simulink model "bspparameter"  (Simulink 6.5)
settings: Solver=ode45  SolverMode=SingleTasking  StartTime=0.0  StopTime=500.0  FixedStep=0.01  RelTol=1e-3
PostLoadFcn:
  | bspparameter_ini
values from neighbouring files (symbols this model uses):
  Konst = 1.15    [bspparameter_ini.m]
  verst = 10    [bspparameter_ini.m]
libraries: simulink x1

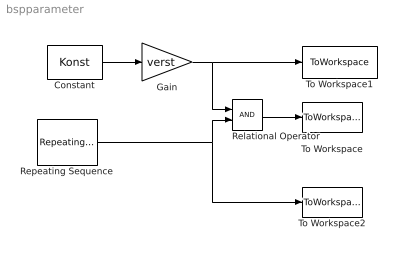
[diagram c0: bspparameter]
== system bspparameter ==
  Constant : Constant  Value=Konst  OutDataType=sfix(16)  ConRadixGroup=Use specified scaling  OutScaling=2^0  SampleTime=inf  FramePeriod=inf
  Gain : Gain  Gain=verst
  Relational Operator : RelationalOperator
  Repeating Sequence : simulink/Sources/Repeating Sequence  SystemSampleTime=-1  rep_seq_t=zeit  rep_seq_y=wiederhol
  To Workspace : ToWorkspace  VariableName=erg  SampleTime=-1  SaveFormat=Array
  To Workspace1 : ToWorkspace  VariableName=verst_Konst  SampleTime=-1  SaveFormat=Array
  To Workspace2 : ToWorkspace  VariableName=repeat  SampleTime=-1  SaveFormat=Array
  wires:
  Relational Operator/1 -> To Workspace/1
  Constant/1 -> Gain/1
  Gain/1 -> Relational Operator/1, To Workspace1/1
  Repeating Sequence/1 -> Relational Operator/2, To Workspace2/1
